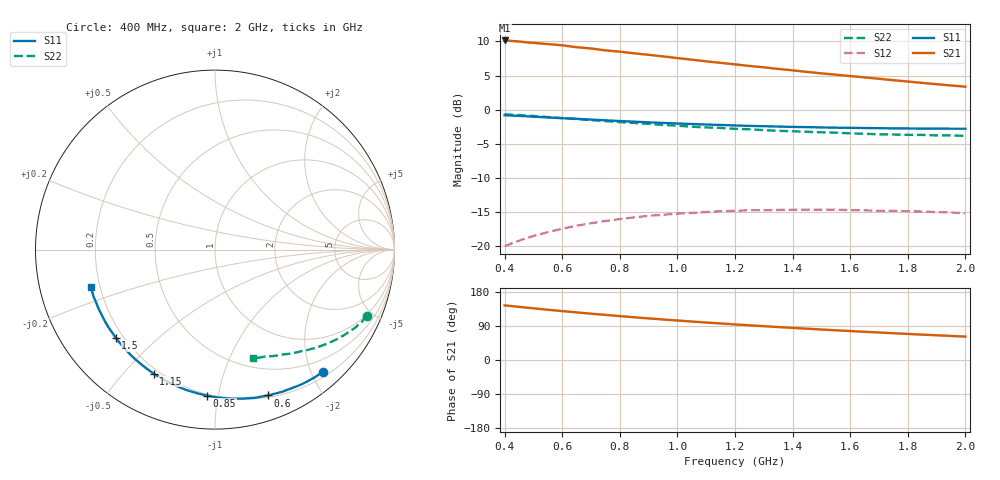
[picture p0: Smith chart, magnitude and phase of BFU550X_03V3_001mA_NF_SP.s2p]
! Filename:  P:\Prog\Test\Noise\ATS_data\Testdata_Net\BFU550X no attenuator noise\BFU550X_APG2013_44_C05_03p3V_001mA_NF_CM01_D.sf
! Date/Time: Fri 26/Jul/2013 14:37:10
! BFU550X_APG2013_44_C05_03p3V_1to10mA_NF_CM01_Bias1_R.sf
! Noise Parameter Data File
! BFU550X_APG2013_44_C05_03p3V_1to10mA_NF_CM01
! Date/time: Wed Jul 24 15:50:55 2013
! freq range =  0.4000 to  2.0000 GHz, 37 points
! bias range =  1.0000 to  9.9950 mA, 5 points
! bias supplies used: 1 1 0 0 0 0
! VAR bias_mode= 1  ! Specify V_out, I_out
! VAR bias_var = 1  ! Bias variable = I_out
! VAR V_out= 3.300000
! VAR I_out= 1.000000
! VAR V_in= 0.777600
! VAR I_in= 0.010901
! Device data file deembeded for feedlines and parallel
! Original file: \BFU550X no attenuator noise\BFU550X_APG2013_44_C05_03p3V_001mA_NF_CM01_R.sf
! Feed-files: PR005V01_100713_Feed1.s2p, PR005V01_100713_Feed2.s2p
! Parallel-file: PR005V01_100713_Par.s2p
# MHz S MA R 50
!  Freq-MHz  S11-mag  S11-arg  S21-mag  S21-arg  S12-mag  S12-arg  S22-mag  S22-arg
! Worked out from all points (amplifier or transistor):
!   37 points, 400 MHz to 2 GHz, reference 50 ohm
!   highest |S21| = 10.2 dB at 400 MHz (marker M1)
!   |S21| within 3 dB of that: start of sweep to 1.086 GHz
!   unconditionally stable (mu >= 1): nowhere
!   at 500 MHz: K = 0.13, MSG = 14.2 dB, |S12| = -18.6 dB
!   at 1.1 GHz: K = 0.27, MSG = 11.1 dB, |S12| = -15.1 dB
!   at 2 GHz: K = 0.49, MSG = 9.3 dB, |S12| = -15.2 dB
!   lowest NFmin = 0.62 dB at 433 MHz
!   S11 on the Smith chart (normalised r, x): 400 MHz: 0.28, -2.19; 600 MHz: 0.22, -1.40; 850 MHz: 0.19, -0.93; 1.15 GHz: 0.18, -0.61; 1.5 GHz: 0.17, -0.37; 2 GHz: 0.16, -0.14
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400  0.9086 -48.6  3.218 144.2  0.09929 59.6  0.9266 -23.6
440  0.9005 -53.1  3.178 141.1  0.1071 57.0  0.9149 -25.5
480  0.8922 -57.4  3.11 137.9  0.1143 54.4  0.9009 -27.5
500  0.8862 -59.6  3.092 136.4  0.1179 53.0  0.8975 -28.6
550  0.8757 -64.9  3.026 132.6  0.1258 49.9  0.8807 -30.9
600  0.8642 -70.1  2.965 129.1  0.1333 47.0  0.8657 -33.1
650  0.8551 -74.9  2.869 125.6  0.1404 44.2  0.8521 -35.0
700  0.8439 -79.8  2.81 122.2  0.1462 41.4  0.8364 -37.2
750  0.8341 -84.3  2.721 119.0  0.152 38.9  0.8233 -38.9
800  0.824 -88.9  2.663 115.8  0.1569 36.4  0.809 -40.8
850  0.8152 -93.2  2.588 112.8  0.1616 34.0  0.7966 -42.5
900  0.8056 -97.5  2.525 109.8  0.1659 31.7  0.7859 -44.0
950  0.7983 -101.6  2.458 106.9  0.1687 29.4  0.7708 -45.9
1050  0.7834 -109.2  2.326 101.5  0.1743 25.3  0.7487 -48.8
1150  0.7709 -116.4  2.203 96.4  0.1794 21.5  0.7333 -51.4
1200  0.7646 -119.9  2.149 93.9  0.1803 19.6  0.7219 -52.9
1350  0.7505 -129.5  1.988 86.9  0.1832 14.5  0.6984 -56.6
1500  0.7394 -138.4  1.845 80.4  0.1842 9.8  0.6813 -60.1
1600  0.7345 -143.9  1.763 76.4  0.1827 7.0  0.6693 -62.6
1750  0.7279 -151.6  1.643 70.6  0.1804 3.1  0.6562 -65.7
1850  0.7248 -156.4  1.57 66.9  0.1785 0.7  0.6515 -67.7
2000  0.7236 -163.2  1.473 61.8  0.1732 -2.5  0.641 -70.8
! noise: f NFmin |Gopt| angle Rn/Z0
400  0.6387  0.6132  28.3  0.3268
460  0.6228  0.5997  38.15  0.2801
600  0.709  0.6482  46.23  0.3542
800  0.7724  0.6197  62.39  0.2959
1000  0.841  0.5969  77.84  0.2686
1200  0.8955  0.6649  94.87  0.2073
1400  0.9617  0.6579  107.1  0.2161
1600  0.8845  0.5823  122.9  0.1181
1800  0.8837  0.5765  135.8  0.0959
2000  1.174  0.6131  145.1  0.0951
